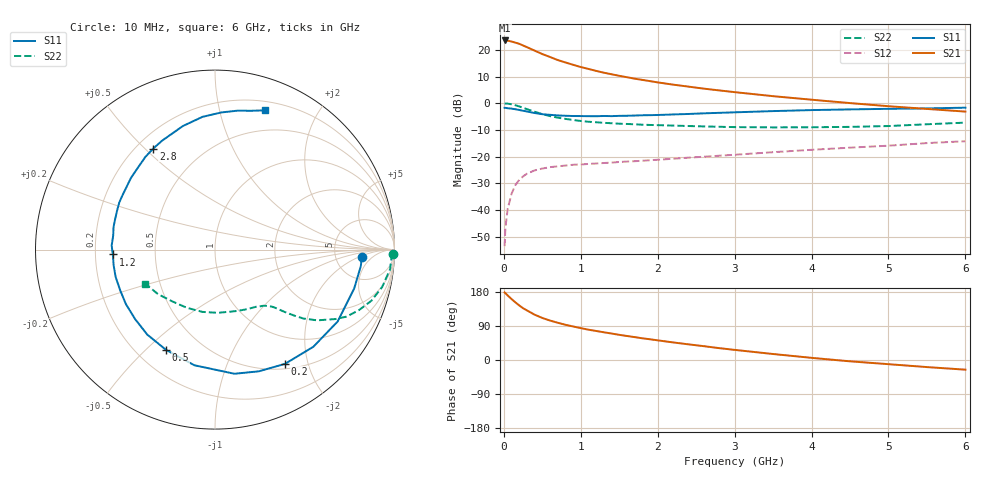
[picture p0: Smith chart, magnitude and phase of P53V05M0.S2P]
! SIEMENS Small Signal Semiconductors
! BFP183
! Si NPN RF Bipolar Junction Transistor in SOT143
! VCE = 3 V  IC = 5 mA
! Common Emitter S-Parameters:  March  1996
# GHz  S  MA  R  50
!  f  S11  S21  S12  S22
! GHz  MAG  ANG  MAG  ANG  MAG  ANG  MAG  ANG
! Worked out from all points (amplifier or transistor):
!   36 points, 10 MHz to 6 GHz, reference 50 ohm
!   highest |S21| = 23.5 dB at 10 MHz (marker M1)
!   |S21| within 3 dB of that: start of sweep to 338 MHz
!   unconditionally stable (mu >= 1): 1.567 GHz to 5.714 GHz
!   at 250 MHz: K = 0.20, MSG = 24.5 dB, |S12| = -27.4 dB
!   at 1.4 GHz: K = 0.94, MSG = 16.5 dB, |S12| = -22.3 dB
!   at 6 GHz: K = 0.95, MSG = 5.5 dB, |S12| = -14.2 dB
!   lowest NFmin = 1.15 dB at 450 MHz
!   S11 on the Smith chart (normalised r, x): 10 MHz: 9.39, -2.44; 200 MHz: 0.57, -1.64; 500 MHz: 0.32, -0.58; 1.2 GHz: 0.27, -0.02; 2.8 GHz: 0.27, +0.53; 6 GHz: 0.29, +1.38
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0.01  0.8187 -3.0  14.96 178.2  0.0021 84.2  0.9928 -1.3
0.02  0.8177 -6.4  14.9 176.5  0.0046 86.5  0.9844 -2.5
0.05  0.8052 -15.6  14.83 170.3  0.0105 83.9  0.9815 -6.4
0.1  0.792 -30.4  14.3 160.9  0.0201 73.6  0.9545 -12.6
0.15  0.7703 -44.6  13.62 152.1  0.0293 67.2  0.9168 -18.1
0.2  0.7467 -58.5  12.96 144.0  0.0367 61.8  0.8702 -22.8
0.25  0.7208 -70.2  12.04 136.7  0.0426 56.3  0.8225 -27.0
0.3  0.7002 -81.1  11.21 130.9  0.0478 51.7  0.7739 -30.0
0.4  0.6546 -100.1  9.658 119.6  0.0551 45.0  0.6925 -34.7
0.5  0.6219 -115.9  8.323 111.0  0.0597 39.7  0.6256 -37.9
0.6  0.6056 -128.5  7.337 104.1  0.0635 36.8  0.5742 -39.8
0.7  0.5901 -138.8  6.432 98.3  0.0656 34.1  0.5367 -41.2
0.8  0.582 -148.5  5.798 93.0  0.0679 32.3  0.5083 -42.3
1.1  0.5715 -171.2  4.382 80.0  0.0729 30.4  0.4494 -45.0
1.2  0.5699 -177.3  4.026 76.6  0.0742 29.7  0.4395 -46.0
1.7  0.5872 158.3  2.882 60.4  0.082 30.4  0.4024 -51.9
2.2  0.6153 139.6  2.227 46.4  0.0911 31.1  0.3807 -59.5
2.8  0.6598 121.4  1.736 31.3  0.1038 31.6  0.3617 -71.4
3.5  0.7112 104.6  1.354 15.8  0.1209 30.5  0.3524 -87.6
4.5  0.7651 87.3  1.005 -3.5  0.147 26.7  0.3602 -115.9
5.5  0.7992 75.4  0.781 -18.7  0.179 21.8  0.4031 -142.0
6  0.8241 70.3  0.696 -25.5  0.194 17.8  0.4327 -154.1
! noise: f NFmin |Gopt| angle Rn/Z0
0.45  1.15  0.25  40  0.26
0.9  1.2  0.25  93  0.22
1.8  1.95  0.32  170  0.13
